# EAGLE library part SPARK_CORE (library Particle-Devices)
Particle/Spark Core WiFi development board footprint (discontinued) Product datasheet: here Design files: here Github : Particle devices library
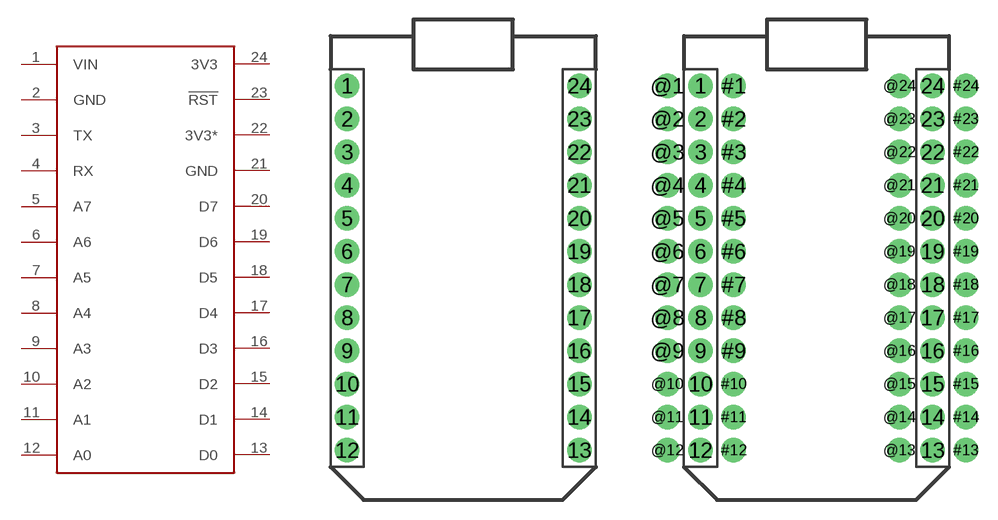
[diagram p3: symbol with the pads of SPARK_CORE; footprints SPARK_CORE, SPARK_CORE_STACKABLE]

Designator prefix -

## SPARK_CORECORE  [SPARK_CORE]
1  VIN  pwr
2  GND  pwr
3  TX
4  RX
5  A7
6  A6
7  A5
8  A4
9  A3
10  A2
11  A1
12  A0
13  D0
14  D1
15  D2
16  D3
17  D4
18  D5
19  D6
20  D7
21  GND  pwr
22  3V3*  pwr
23  !RST
24  3V3  pwr

## SPARK_CORE  [SPARK_CORE_STACKABLE]
1  VIN  pwr
2  GND  pwr
3  TX
4  RX
5  A7
6  A6
7  A5
8  A4
9  A3
10  A2
11  A1
12  A0
13  D0
14  D1
15  D2
16  D3
17  D4
18  D5
19  D6
20  D7
21  GND  pwr
22  3V3*  pwr
23  !RST
24  3V3  pwr
#1  VIN  pwr
#2  GND  pwr
#3  TX
#4  RX
#5  A7
#6  A6
#7  A5
#8  A4
#9  A3
#10  A2
#11  A1
#12  A0
#13  D0
#14  D1
#15  D2
#16  D3
#17  D4
#18  D5
#19  D6
#20  D7
#21  GND  pwr
#22  3V3*  pwr
#23  !RST
#24  3V3  pwr
@1  VIN  pwr
@2  GND  pwr
@3  TX
@4  RX
@5  A7
@6  A6
@7  A5
@8  A4
@9  A3
@10  A2
@11  A1
@12  A0
@13  D0
@14  D1
@15  D2
@16  D3
@17  D4
@18  D5
@19  D6
@20  D7
@21  GND  pwr
@22  3V3*  pwr
@23  !RST
@24  3V3  pwr

## Footprint SPARK_CORE (pad centres in mm)
drill 1.016 pad 1.88: 1 -8.89,13.97; 2 -8.89,11.43; 3 -8.89,8.89; 4 -8.89,6.35; 5 -8.89,3.81; 6 -8.89,1.27; 7 -8.89,-1.27; 8 -8.89,-3.81; 9 -8.89,-6.35; 10 -8.89,-8.89; 11 -8.89,-11.43; 12 -8.89,-13.97; 13 8.89,-13.97; 14 8.89,-11.43; 15 8.89,-8.89; 16 8.89,-6.35; 17 8.89,-3.81; 18 8.89,-1.27; 19 8.89,1.27; 20 8.89,3.81; 21 8.89,6.35; 22 8.89,8.89; 23 8.89,11.43; 24 8.89,13.97

## Footprint SPARK_CORE_STACKABLE (pad centres in mm)
drill 1.016 pad 1.88: 1 -8.89,13.97; 2 -8.89,11.43; 3 -8.89,8.89; 4 -8.89,6.35; 5 -8.89,3.81; 6 -8.89,1.27; 7 -8.89,-1.27; 8 -8.89,-3.81; 9 -8.89,-6.35; 10 -8.89,-8.89; 11 -8.89,-11.43; 12 -8.89,-13.97; 13 8.89,-13.97; 14 8.89,-11.43; 15 8.89,-8.89; 16 8.89,-6.35; 17 8.89,-3.81; 18 8.89,-1.27; 19 8.89,1.27; 20 8.89,3.81; 21 8.89,6.35; 22 8.89,8.89; 23 8.89,11.43; 24 8.89,13.97; #1 -6.35,13.97; #2 -6.35,11.43; #3 -6.35,8.89; #4 -6.35,6.35; #5 -6.35,3.81; #6 -6.35,1.27; #7 -6.35,-1.27; #8 -6.35,-3.81; #9 -6.35,-6.35; #10 -6.35,-8.89; #11 -6.35,-11.43; #12 -6.35,-13.97; #13 11.43,-13.97; #14 11.43,-11.43; #15 11.43,-8.89; #16 11.43,-6.35; #17 11.43,-3.81; #18 11.43,-1.27; #19 11.43,1.27; #20 11.43,3.81; #21 11.43,6.35; #22 11.43,8.89; #23 11.43,11.43; #24 11.43,13.97; @1 -11.43,13.97; @2 -11.43,11.43; @3 -11.43,8.89; @4 -11.43,6.35; @5 -11.43,3.81; @6 -11.43,1.27; @7 -11.43,-1.27; @8 -11.43,-3.81; @9 -11.43,-6.35; @10 -11.43,-8.89; @11 -11.43,-11.43; @12 -11.43,-13.97; @13 6.35,-13.97; @14 6.35,-11.43; @15 6.35,-8.89; @16 6.35,-6.35; @17 6.35,-3.81; @18 6.35,-1.27; @19 6.35,1.27; @20 6.35,3.81; @21 6.35,6.35; @22 6.35,8.89; @23 6.35,11.43; @24 6.35,13.97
